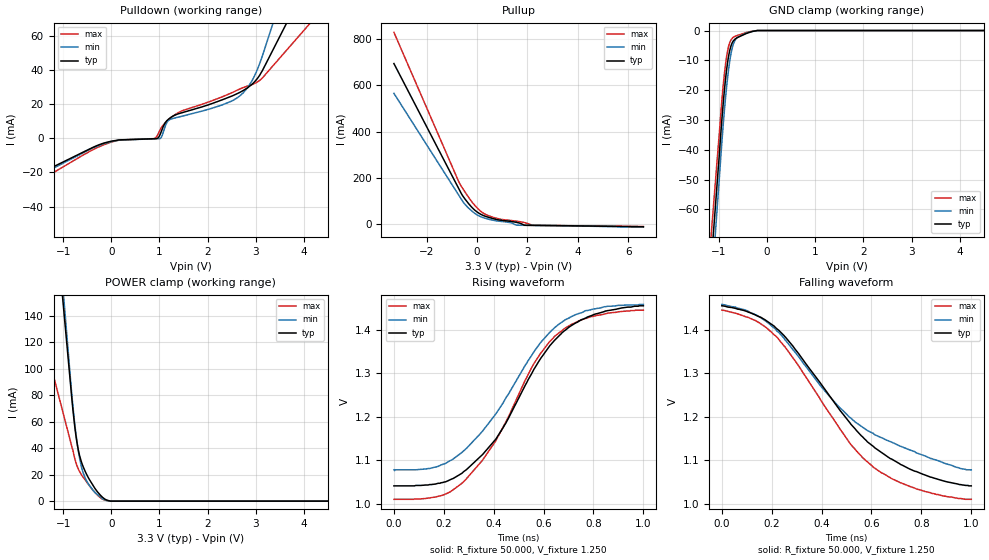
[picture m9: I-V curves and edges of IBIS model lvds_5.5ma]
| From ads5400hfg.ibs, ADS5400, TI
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[Model]   lvds_5.5ma
Model_type 3-state
Vref=1.250E+00
Rref=5.000E+01
Cref=0.000E+00
Vmeas=1.250E+00
C_comp   4.960E-13   4.830E-13   5.040E-13
[Voltage Range]   3.300E+00   3.000E+00   3.600E+00
[POWER Clamp Reference]   3.300E+00   3.000E+00   3.600E+00
[GND Clamp Reference]   0.000E+00   0.000E+00   0.000E+00
[Pullup Reference]   3.300E+00   3.000E+00   3.600E+00
[Pulldown Reference]   0.000E+00   0.000E+00   0.000E+00
[Temperature Range]   25   100   -40
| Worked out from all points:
|   slope of the pulldown table from 0 to 0.495 V, typ, clamps not added: 458 ohm
|   slope of the pullup table from 0 to 0.495 V, typ, clamps not added: 20.3 ohm
|   GND clamp passes 1 mA (typ) near -0.43 V on its own axis
|   POWER clamp passes 1 mA (typ) near -0.11 V on its own axis
|   rising waveform, R_fixture 50.000, V_fixture 1.250: 20-80 % time 267ps typ, 271ps min, 254ps max; typ from 1.04 V to 1.46 V
|   falling waveform, R_fixture 50.000, V_fixture 1.250: 20-80 % time 354ps typ, 384ps min, 325ps max; typ from 1.46 V to 1.04 V
[GND Clamp]
-3.3V     -538.5mA   -570.2mA   -501.4mA
-1.02V    -47.23mA   -55.53mA   -39.73mA
-920mV    -25.89mA   -33.13mA   -19.73mA
-880mV    -18.79mA   -25.37mA   -13.44mA
-840mV    -12.93mA   -18.63mA   -8.563mA
-800mV    -8.532mA   -12.99mA   -5.283mA
-760mV    -5.622mA   -8.585mA   -3.428mA
-720mV    -3.947mA   -5.521mA   -2.501mA
-660mV    -2.791mA   -3.07mA    -1.891mA
-440mV    -1.048mA   -875.8uA   -712.4uA
-200mV    0A         0A         0A
6.6V      0A         0A         0A
[Power Clamp]
-3.3V     1.067A     1.164A     389.5mA
-900mV    109.4mA    115.3mA    52.41mA
-820mV    77.51mA    80.37mA    41.17mA
-740mV    50.89mA    52.41mA    29.74mA
-680mV    37.73mA    36.94mA    23.88mA
-620mV    29.53mA    25.85mA    19.94mA
-540mV    22.27mA    17.31mA    15.99mA
-460mV    16.62mA    12.14mA    11.86mA
-320mV    8.591mA    5.91mA     5.729mA
-180mV    2.808mA    1.892mA    1.433mA
-20mV     0A         0A         0A
6.6V      0A         0A         0A
[Pullup]
-3.3V     694.5mA    565.5mA    829.8mA
-720mV    151.5mA    123.4mA    181.4mA
-520mV    114mA      90.22mA    145.5mA
-300mV    83.35mA    64.85mA    109.8mA
-100mV    60.68mA    46.56mA    81.92mA
160mV     40.98mA    30.74mA    53.49mA
820mV     18.17mA    12.64mA    23.18mA
1.34V     10.81mA    5.154mA    14.99mA
1.58V     6.473mA    -5.361mA   11.7mA
1.88V     -5.396mA   -5.953mA   5.852mA
2.22V     -6.243mA   -6.333mA   -5.859mA
6.6V      -12.24mA   -13.96mA   -11.25mA
[Pulldown]
-3.3V     -45.72mA   -48.03mA   -55.2mA
-380mV    -5.282mA   -5.61mA    -6.649mA
160mV     -932.9uA   -1.035mA   -1.068mA
900mV     -217.3uA   -282.4uA   -151.7uA
960mV     19.75uA    -228.3uA   1.796mA
1.04V     4.073mA    618.8uA    6.29mA
1.12V     9.131mA    7.106mA    9.112mA
1.28V     13.08mA    11.66mA    13.04mA
2.52V     24.99mA    22.13mA    26.95mA
2.92V     31.63mA    33.58mA    31.48mA
3.16V     40.9mA     50.23mA    36.12mA
6.6V      231.5mA    349.5mA    147.4mA
[Rising Waveform]
R_fixture = 50.000
V_fixture = 1.250
V_fixture_min = 1.250
V_fixture_max = 1.250
|  time   V(typ)   V(min)   V(max)
0s        1.041V     1.078V     1.01V
165ps     1.045V     1.084V     1.015V
225ps     1.055V     1.099V     1.027V
280ps     1.074V     1.122V     1.051V
410ps     1.15V      1.208V     1.147V
562.5ps   1.311V     1.351V     1.324V
625ps     1.364V     1.395V     1.374V
682.5ps   1.398V     1.422V     1.403V
807.5ps   1.437V     1.449V     1.433V
1ns       1.456V     1.459V     1.446V
[Falling Waveform]
R_fixture = 50.000
V_fixture = 1.250
V_fixture_min = 1.250
V_fixture_max = 1.250
|  time   V(typ)   V(min)   V(max)
0s        1.456V     1.459V     1.446V
137.5ps   1.434V     1.435V     1.421V
222.5ps   1.402V     1.397V     1.383V
285ps     1.363V     1.355V     1.336V
465ps     1.222V     1.226V     1.18V
517.5ps   1.183V     1.197V     1.136V
607.5ps   1.132V     1.162V     1.084V
772.5ps   1.075V     1.12V      1.036V
897.5ps   1.051V     1.092V     1.017V
1ns       1.041V     1.078V     1.01V
[Ramp]
dV/dt_f   2.4900E-01/3.9609E-10   2.2860E-01/5.1500E-10   2.6160E-01/3.5422E-10
dV/dt_r   2.4900E-01/2.8190E-10   2.2860E-01/2.7460E-10   2.6160E-01/2.6100E-10
R_load = 50
